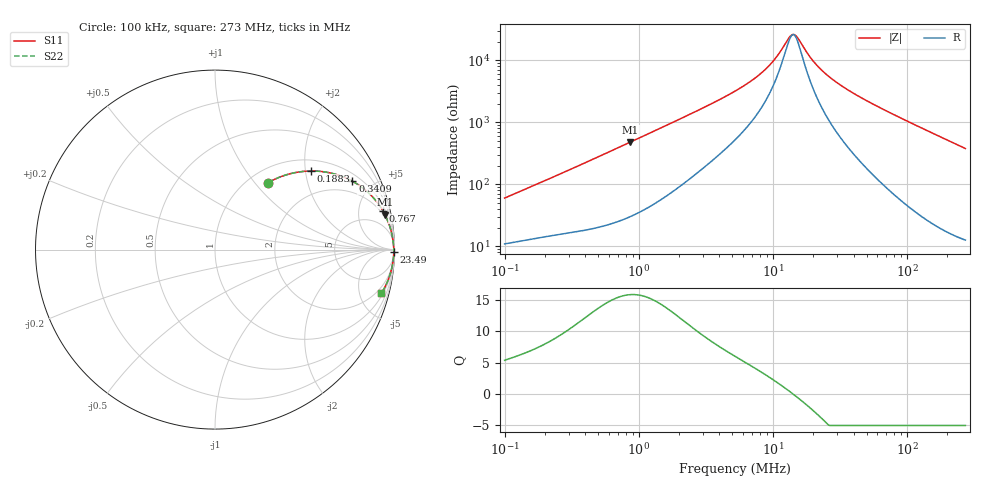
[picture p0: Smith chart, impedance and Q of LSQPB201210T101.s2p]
! LSQPB201210T101  S-PARAMETER MODEL  ( General Type )
! Model Generated by TAIYO YUDEN Corporation (http://www.ty-top.com)
! Version 2.0
! TAIYO YUDEN Control No. 100810NF18SB-HKC
! Copyright(c) 2007 TAIYO YUDEN CO.,LTD. All Rights Reserved.
! Product Description (link to TY-COMPAS)
! https://ds.yuden.co.jp/TYCOMPAS/or/detail?pn=LSQPB201210T101M&u=M
! Products Name : Inductors
! Characteristics :
!  Inductance : 100 uH , SRF(min) : 6.0 MHz , DC Resistance(max) : 10.01 Ohm
!  Rated Current : Saturation :85 mA , Temp Rise : 85 mA (40 degC)
!  Case Size : 2.0 x 1.25 / 0.079 x 0.049 [mm/inch] , Thickness : 1.0 / 0.04 [mm/inch]
!  (Conditions: Temperature = 25 degC , DC Bias Current/Voltage = 0A / 0V)
! External Node Assignments :
!  1  o---GGG---o  2
! GND o---------o GND
! Frequency Range : 0.1MHz  -  272.98108MHz  [ 402 STEP ]
# MHz S RI R 50
! Freq[MHz].  S11 Real  S11 Imag  S21 Real  S21 Imag  S12 Real  S12 Imag  S22 Real  S22 Imag
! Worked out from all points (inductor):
!   401 points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, 100 kHz to 273 MHz, reference 50 ohm
!   read as one part in series: L = 92.6 uH near 104 kHz
!   highest Q = 15.9 at 863.7 kHz (marker M1), where L = 87.8 uH
!   self-resonance near 14.05 MHz
!   S11 on the Smith chart (normalised r, x): 100 kHz: 1.22, +1.18; 188.3 kHz: 1.28, +2.15; 340.9 kHz: 1.34, +3.80; 767 kHz: 1.54, +8.47; 23.49 MHz: open; 273 MHz: 1.25, -7.54
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0.1  0.2971 0.3735  0.7029 -0.3735  0.7029 -0.3735  0.2971 0.3735
0.188317  0.5352 0.438  0.4648 -0.438  0.4648 -0.438  0.5352 0.438
0.340879  0.7652 0.3812  0.2348 -0.3812  0.2348 -0.3812  0.7652 0.3812
0.376316  0.796 0.3627  0.204 -0.3627  0.204 -0.3627  0.796 0.3627
0.52673  0.8787 0.2927  0.1213 -0.2927  0.1213 -0.2927  0.8787 0.2927
0.767015  0.935 0.2167  0.065 -0.2167  0.065 -0.2167  0.935 0.2167
0.863667  0.9467 0.1953  0.0533 -0.1953  0.0533 -0.1953  0.9467 0.1953
1.416134  0.9758 0.1232  0.0242 -0.1232  0.0242 -0.1232  0.9758 0.1232
3.250112  0.9911 0.0532  0.00892 -0.0532  0.00892 -0.0532  0.9911 0.0532
5.329134  0.994 0.03  0.00601 -0.03  0.00601 -0.03  0.994 0.03
7.169875  0.995 0.0196  0.00498 -0.0196  0.00498 -0.0196  0.995 0.0196
9.090663  0.9956 0.0123  0.00441 -0.0123  0.00441 -0.0123  0.9956 0.0123
10.86197  0.9959 0.00727  0.00411 -0.00727  0.00411 -0.00727  0.9959 0.00727
13.23768  0.9961 0.00186  0.00388 -0.00186  0.00388 -0.00186  0.9961 0.00186
14.04698  0.9962 0.000251  0.00384 -0.000251  0.00384 -0.000251  0.9962 0.000251
15.20352  0.9962 -0.0019  0.00379 0.0019  0.00379 0.0019  0.9962 -0.0019
19.66158  0.9963 -0.00907  0.00374 0.00907  0.00374 0.00907  0.9963 -0.00907
23.49262  0.9962 -0.0144  0.00382 0.0144  0.00382 0.0144  0.9962 -0.0144
36.30101  0.9955 -0.0297  0.00445 0.0297  0.00445 0.0297  0.9955 -0.0297
73.9896  0.9914 -0.0685  0.00855 0.0685  0.00855 0.0685  0.9914 -0.0685
144.9579  0.9762 -0.1357  0.0238 0.1357  0.0238 0.1357  0.9762 -0.1357
272.9811  0.9273 -0.2435  0.0727 0.2435  0.0727 0.2435  0.9273 -0.2435
